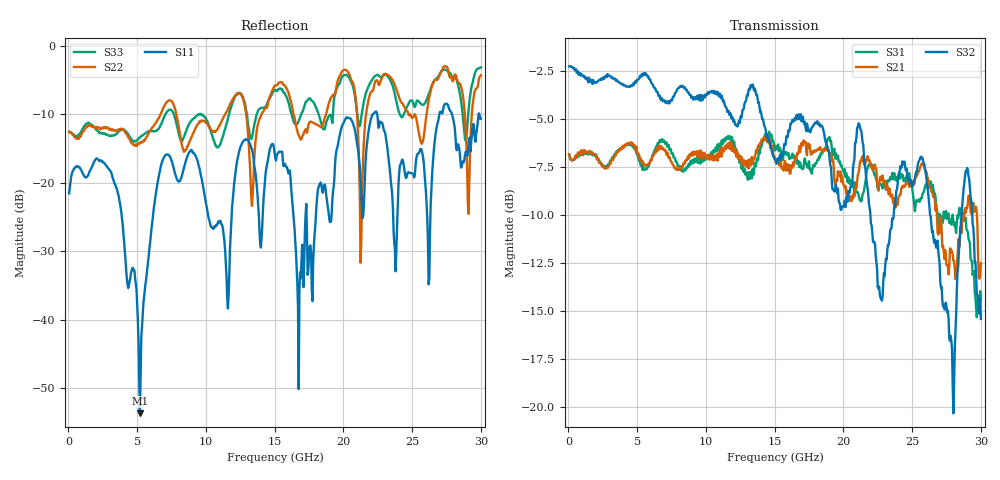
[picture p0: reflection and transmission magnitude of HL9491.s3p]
! 9/10/2021 10:14:16 AM
! H:\PRODUCTION_DATA\TEMP_S3P.S3P
! CHANNEL.1
! TR.MEASUREMENT
! CORRECTED.DATA
# GHZ S RI R 50.0
! FREQ.GHZ  S11RE  S11IM  S12RE  S12IM  S13RE  S13IM
!  S21RE  S21IM  S22RE  S22IM  S23RE  S23IM
!  S31RE  S31IM  S32RE  S32IM  S33RE  S33IM
!; PortSelection: Port_123
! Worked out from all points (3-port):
!   600 points, 50 MHz to 30 GHz, reference 50 ohm
!   strongest paths, dB at 50 MHz, 7.55 GHz, 15.05 GHz, 22.55 GHz, 30 GHz:
!     S32: -2.3, -4.0, -7.2, -13.8, -15.4
!     S21: -6.8, -7.3, -7.2, -8.7, -12.5
!     S31: -6.8, -6.8, -6.6, -8.7, -14.4
!   lowest |S11| = -53.7 dB at 5.2 GHz (marker M1), VSWR 1.00, Z = 50.2 - j0.00729 ohm
!   |S11| at or under -10 dB: start of sweep to 22.14 GHz; 22.46 GHz to 26.98 GHz (4.524 GHz wide, 18.3 % of centre); 27.9 GHz to 29.84 GHz (1.942 GHz wide, 6.73 % of centre)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
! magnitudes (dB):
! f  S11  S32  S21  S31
! 50 MHz  -21.6  -2.3  -6.8  -6.8
! 3.1 GHz  -18.4  -2.8  -7.3  -7.2
! 5.2 GHz  -53.7  -2.8  -7.1  -7.1
! 7 GHz  -16.1  -4.1  -6.7  -6.2
! 11.55 GHz  -36.8  -4.6  -6.3  -6.0
! 15.05 GHz  -16.4  -7.2  -7.2  -6.6
! 16.75 GHz  -50.1  -4.8  -6.7  -7.2
! 20.2 GHz  -10.5  -9.2  -8.9  -7.8
! 21.3 GHz  -21.5  -5.6  -7.2  -9.3
! 30 GHz  -10.7  -15.4  -12.5  -14.4
